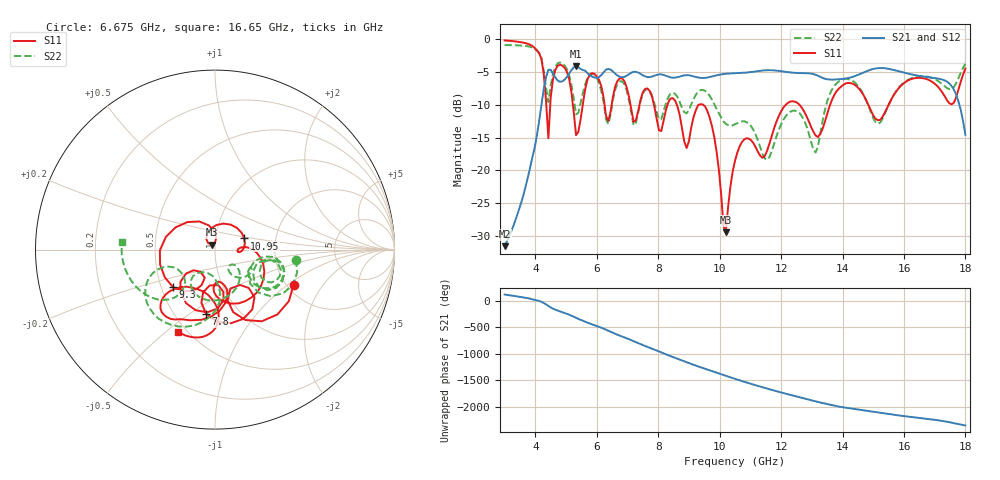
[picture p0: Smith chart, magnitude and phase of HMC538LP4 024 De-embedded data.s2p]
! Chelmsford, MA 01824
! http://www.hittite.com
! Tel: 978-250-3343
! Fax: 978-250-3373
! Device  :  HMC538LP4
! Description:  600 Analog Phase Shifter
! Frequency  :  6.0 GHz - 15.0 GHz
! Package  :  LP4  - 4x4 mm Quad Flatpack No-Lead (QFN) Plastic Package: 24 pin
! Ports  :  2 RF, 1 DC
!  Pin  3  = Rfin  = Port 1
!  Pin  16  = Rfout = Port 2
!  pin  21  = vCTL
! Voltages:  VCTL  = 0 to 5.0 Volts
! Currents :  Vb(V)  Vd(V)  Ib(mA)  Id(mA)
!  0.00  2.40  0.000000	0.472386
! Data:  The device was measured on evaluation board 111296-1.
!  Data was collected using a calibrated network analyzer.
!  The evaluation circuit board was modeled and simulated.This was use
!  to removed the evaluation board circuit from the measured data.
!  The reference plane is the center of the package pin.
! Misc:  Lot #
!Date Measured:  03 - 11 -2009
! Date:  03 - 17 -2009
! Note:
!  Hittite Microwave supplies this data as a sample of measured data at the
!  package pin for this package product.  Your particular data for this product
!  may vary.
!  Data was taken at 25 degrees C.
!  Hittite Microwave reserves the right to change this data at anytime.
# MHz S MA R 50
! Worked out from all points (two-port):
!   201 points, 3 GHz to 18 GHz, reference 50 ohm
!   highest |S21| = -4.12 dB at 5.325 GHz (marker M1); lowest = -31.5 dB at 3 GHz (marker M2)
!   |S21| within 3 dB of the highest: 4.295 GHz to 17.54 GHz (13.25 GHz wide, 121 % of centre)
!   lowest |S11| = -29.4 dB at 10.2 GHz (marker M3), VSWR 1.07, Z = 48 + j2.68 ohm
!   |S11| at or under -10 dB: 8.604 GHz to 9.333 GHz (728.5 MHz wide, 8.12 % of centre); 9.456 GHz to 12.16 GHz (2.7 GHz wide, 25 % of centre); 12.59 GHz to 13.6 GHz (1.003 GHz wide, 7.66 % of centre)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
!   |S22| runs from -18.4 to -0.9 dB; largest |S21 - S12| = 0.0026
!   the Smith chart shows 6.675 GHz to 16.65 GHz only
!   S11 on the Smith chart (normalised r, x): 6.675 GHz: 2.18, -1.10; 7.8 GHz: 0.71, -0.58; 9.3 GHz: 0.58, -0.27; 10.95 GHz: 1.38, +0.18; 16.65 GHz: 0.45, -0.55
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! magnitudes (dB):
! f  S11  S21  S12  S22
! 3 GHz  -0.2  -31.5  -31.5  -0.9
! 4.125 GHz  -2.2  -12.5  -12.4  -2.2
! 4.425 GHz  -15.1  -4.7  -4.7  -9.6
! 4.8 GHz  -3.9  -6.5  -6.5  -3.6
! 5.325 GHz  -14.6  -4.1  -4.1  -11.5
! 5.55 GHz  -9.8  -4.7  -4.7  -8.2
! 5.925 GHz  -5.3  -5.9  -5.9  -5.4
! 6.375 GHz  -12.5  -4.6  -4.6  -13.0
! 6.675 GHz  -6.4  -5.6  -5.6  -6.8
! 7.2 GHz  -12.6  -5.0  -5.0  -13.1
! 7.8 GHz  -8.8  -5.7  -5.7  -8.6
! 8.025 GHz  -13.9  -5.4  -5.4  -12.2
! 9.3 GHz  -10.1  -5.9  -5.9  -8.0
! 9.75 GHz  -13.3  -5.7  -5.7  -9.2
! 10.2 GHz  -29.4  -5.3  -5.3  -12.9
! 10.5 GHz  -18.5  -5.2  -5.2  -13.0
! 10.95 GHz  -15.2  -5.1  -5.1  -12.9
! 13.05 GHz  -14.1  -5.3  -5.4  -16.8
! 13.88 GHz  -7.6  -6.1  -6.1  -6.5
! 15.53 GHz  -9.8  -4.6  -4.6  -9.8
! 16.65 GHz  -6.0  -5.7  -5.8  -5.7
! 18 GHz  -4.5  -14.6  -14.6  -3.8
